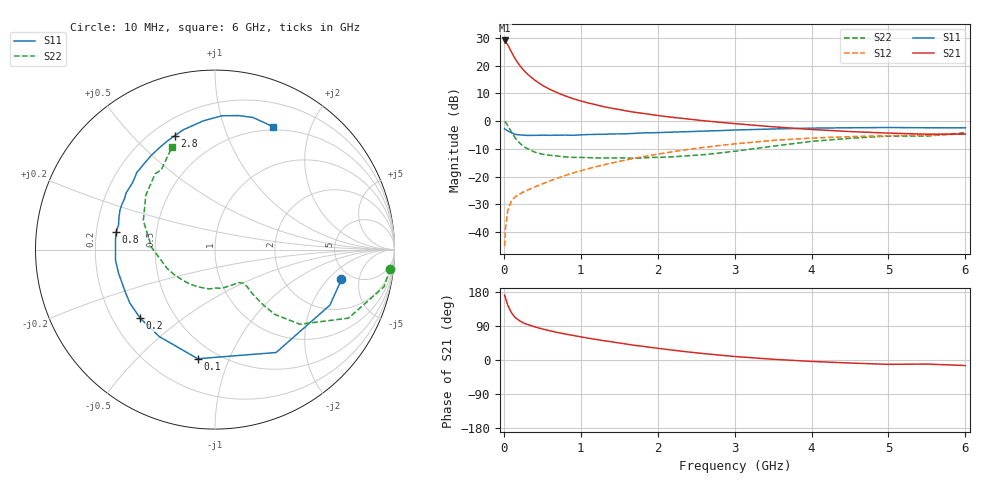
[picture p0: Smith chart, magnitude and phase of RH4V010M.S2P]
! SIEMENS Small Signal Semiconductors
! BFR106
! Si NPN RF Bipolar Junction Transistor in SOT23
! VCE = 4 V  IC = 10 mA
! Common Emitter S-Parameters:  August  1996
# GHz  S  MA  R  50
!  f  S11  S21  S12  S22
! GHz  MAG  ANG  MAG  ANG  MAG  ANG  MAG  ANG
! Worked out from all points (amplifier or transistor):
!   36 points, 10 MHz to 6 GHz, reference 50 ohm
!   highest |S21| = 29.0 dB at 10 MHz (marker M1)
!   |S21| within 3 dB of that: start of sweep to 77.04 MHz
!   unconditionally stable (mu >= 1): 488 MHz to 2.068 GHz; 5.198 GHz to end of sweep
!   at 250 MHz: K = 0.71, MSG = 22.1 dB, |S12| = -25.6 dB
!   at 1.4 GHz: K = 1.09, MAG = 8.0 dB, |S12| = -15.1 dB
!   at 6 GHz: K = 1.01, MAG = -0.7 dB, |S12| = -4.6 dB
!   S11 on the Smith chart (normalised r, x): 10 MHz: 4.14, -2.90; 100 MHz: 0.40, -0.77; 200 MHz: 0.32, -0.36; 800 MHz: 0.28, +0.08; 2.8 GHz: 0.29, +0.67; 6 GHz: 0.47, +1.48
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0.01  0.7241 -13.3  28.28 171.3  0.0056 83.1  0.9817 -6.3
0.02  0.7111 -25.8  27.57 164.5  0.0111 78.2  0.9642 -12.4
0.05  0.6668 -59.3  23.67 144.8  0.0244 63.6  0.8358 -27.2
0.1  0.6156 -99.0  17.37 124.5  0.0373 51.6  0.63 -41.3
0.15  0.5755 -122.7  13.03 111.6  0.0435 46.9  0.4915 -47.3
0.2  0.5655 -137.4  10.34 104.2  0.0483 46.6  0.4103 -48.9
0.25  0.5602 -147.9  8.44 98.2  0.0525 47.3  0.3538 -49.4
0.3  0.5526 -155.3  7.147 94.2  0.0565 49.0  0.3216 -49.7
0.4  0.5532 -166.2  5.476 87.6  0.0651 52.1  0.2767 -49.2
0.5  0.5575 -173.8  4.408 81.9  0.074 55.1  0.2535 -49.1
0.6  0.5544 179.9  3.717 77.1  0.0839 57.0  0.2427 -50.2
0.7  0.557 174.2  3.217 72.5  0.0941 59.2  0.2341 -52.3
0.8  0.5599 170.1  2.833 68.6  0.1053 60.0  0.2264 -54.3
1.1  0.573 157.6  2.115 57.5  0.1392 61.8  0.2196 -63.6
1.3  0.5785 150.6  1.818 50.9  0.1633 61.6  0.2165 -70.7
1.6  0.5915 140.9  1.518 41.8  0.2008 60.3  0.2164 -83.9
2.2  0.6335 124.3  1.165 25.9  0.282 54.5  0.2276 -114.2
2.8  0.673 109.5  0.955 13.0  0.3624 46.0  0.2666 -148.5
3.5  0.7206 95.1  0.79 1.9  0.4489 34.5  0.3537 178.0
4.5  0.7582 80.0  0.648 -8.0  0.5246 17.2  0.4903 141.8
5.5  0.7584 68.3  0.58 -10.7  0.5569 6.0  0.5363 123.9
6  0.756 64.5  0.584 -14.6  0.5867 -1.8  0.619 112.8
